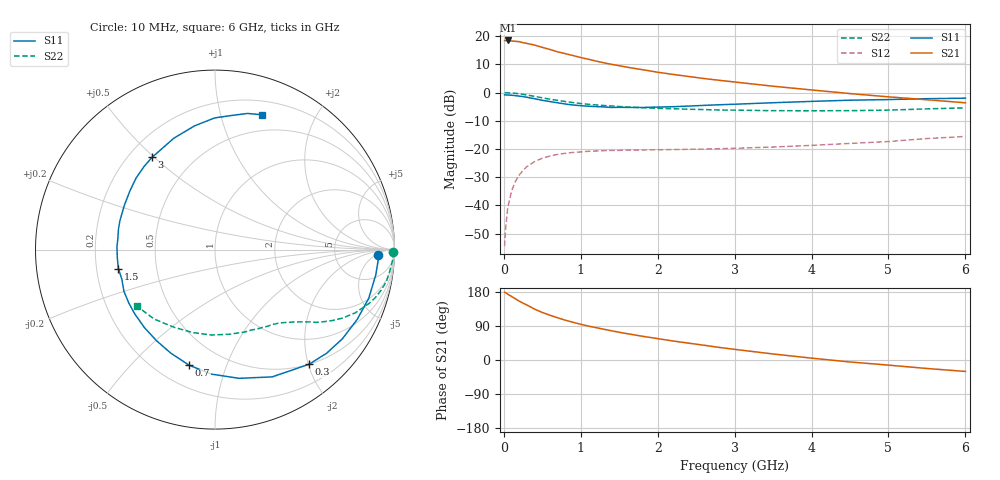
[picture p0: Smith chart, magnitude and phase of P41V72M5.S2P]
! SIEMENS Small Signal Semiconductors
! BFP182
! Si NPN RF Bipolar Junction Transistor in SOT143
! VCE = 1.75 V  IC = 2.5 mA
! Common Emitter S-Parameters:  March  1996
# GHz  S  MA  R  50
!  f  S11  S21  S12  S22
! GHz  MAG  ANG  MAG  ANG  MAG  ANG  MAG  ANG
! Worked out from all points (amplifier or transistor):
!   36 points, 10 MHz to 6 GHz, reference 50 ohm
!   highest |S21| = 18.5 dB at 50 MHz (marker M1)
!   |S21| within 3 dB of that: start of sweep to 573.4 MHz
!   unconditionally stable (mu >= 1): 1.996 GHz to end of sweep
!   at 250 MHz: K = 0.15, MSG = 22.6 dB, |S12| = -27.6 dB
!   at 1.4 GHz: K = 0.75, MSG = 15.3 dB, |S12| = -20.5 dB
!   at 6 GHz: K = 1.00, MAG = 5.8 dB, |S12| = -15.6 dB
!   S11 on the Smith chart (normalised r, x): 10 MHz: 19, -7; 300 MHz: 0.50, -2.01; 700 MHz: 0.33, -0.75; 1.5 GHz: 0.29, -0.09; 3 GHz: 0.29, +0.49; 6 GHz: 0.33, +1.36
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0.01  0.9112 -1.9  8.31 179.0  0.0019 81.8  0.9944 -0.7
0.02  0.9111 -3.6  8.33 178.1  0.0035 83.0  0.9934 -1.4
0.05  0.9068 -8.9  8.394 173.8  0.009 88.0  0.9914 -3.5
0.1  0.8985 -17.6  8.228 167.7  0.018 79.6  0.9807 -7.1
0.2  0.8664 -35.0  7.995 155.4  0.0346 70.1  0.9525 -13.8
0.3  0.826 -50.7  7.443 145.0  0.0488 62.0  0.9081 -19.4
0.4  0.7775 -65.8  6.947 134.2  0.06 54.2  0.8579 -24.2
0.5  0.7296 -79.4  6.335 125.4  0.0687 47.9  0.8085 -28.1
0.6  0.694 -91.7  5.806 118.1  0.0752 42.6  0.7647 -31.1
0.7  0.6597 -102.7  5.272 111.3  0.0805 38.7  0.7276 -33.5
0.8  0.627 -113.2  4.893 105.0  0.0839 34.8  0.6944 -35.7
0.9  0.6032 -122.7  4.533 99.5  0.0871 31.7  0.6643 -37.3
1.1  0.5732 -141.0  3.897 89.4  0.0913 27.1  0.6212 -40.4
1.3  0.5581 -155.4  3.373 81.1  0.0935 23.4  0.5906 -43.1
1.5  0.5488 -168.9  2.993 73.1  0.0946 21.0  0.567 -45.7
1.8  0.545 172.9  2.549 62.6  0.0962 19.1  0.5401 -49.5
2.2  0.5623 153.9  2.099 50.2  0.0978 17.4  0.5181 -55.5
3  0.6222 124.3  1.541 28.1  0.1031 17.3  0.4886 -69.9
3.5  0.6615 110.3  1.297 15.9  0.1086 17.8  0.4783 -80.4
4.5  0.7335 90.2  0.961 -5.2  0.1257 18.2  0.4787 -105.1
5.5  0.7798 76.6  0.747 -22.4  0.1535 16.6  0.5146 -131.2
6  0.7965 70.6  0.66 -30.2  0.1668 13.3  0.5365 -143.9
